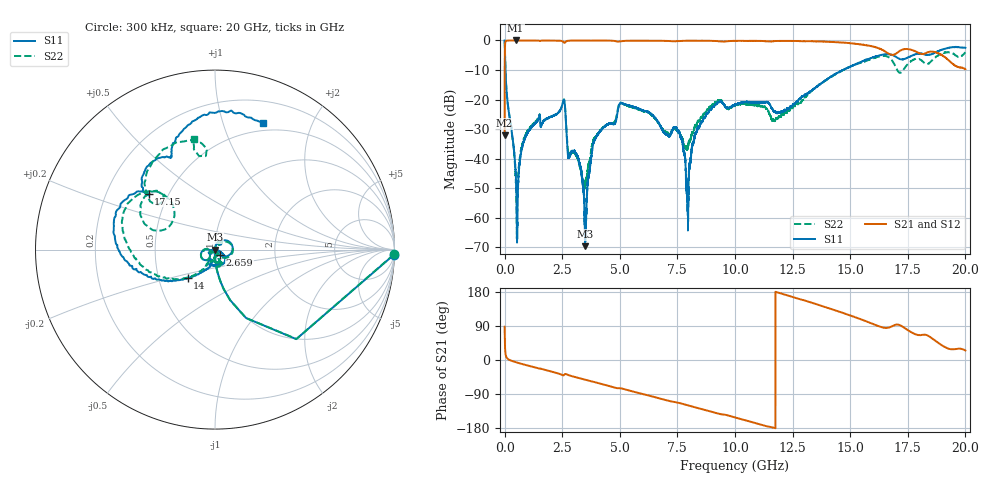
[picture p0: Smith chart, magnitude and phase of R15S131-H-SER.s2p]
!{R15S131}
!Johanson Technology Inc.
!www.johansontechnology.com
!Test Board Conditions:
!Substrate Type  RO4350B
!Substrate Thickness  20 mil
!Substrate Dk  3.66
!TL Type: GCPW
!TL Trace Width  34 mil
!TL Gap  10 mil
!Electrode orientation  Horizontal
!DUT TOPOLOGY	SERIES
!Mounting Pad LxW  26x52 mil
! Created Sat Feb  6 14:11:45 2021
# hz S ma R 50
! 2 Port Network Data from SP1.SP block
! freq  magS11  angS11  magS21  angS21  magS12  angS12  magS22  angS22
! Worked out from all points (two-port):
!   20001 points, 300 kHz to 20 GHz, reference 50 ohm
!   highest |S21| = 0.00 dB at 477.3 MHz (marker M1); lowest = -32.2 dB at 300 kHz (marker M2)
!   |S21| within 3 dB of the highest: 12.21 MHz to 16.35 GHz (16.34 GHz wide, 200 % of centre); 17.31 GHz to 17.57 GHz (265 MHz wide, 1.52 % of centre)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
!   lowest |S11| = -69.6 dB at 3.491 GHz (marker M3), VSWR 1.00, Z = 50 + j0.0294 ohm
!   |S11| at or under -10 dB: 36.21 MHz to 14.67 GHz (14.63 GHz wide, 199 % of centre); 14.66745 GHz to 14.67174 GHz (4.29 MHz wide, 0.0292 % of centre); 14.6865 GHz to 14.69163 GHz (5.126 MHz wide, 0.0349 % of centre)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
!   |S22| runs from -67.1 to 0.0 dB; largest |S21 - S12| = 0.018
!   S11 on the Smith chart (normalised r, x): 300 kHz: 6, -70; 2.659 GHz: 1.06, -0.07; 14 GHz: 0.70, -0.23; 17.15 GHz: 0.39, +0.32; 20 GHz: 0.42, +1.36
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300000  0.9976 -1.6  0.02468 87.8  0.02476 88.3  0.9963 -1.6
1.063e8  0.1103 -84.8  0.9932 4.9  0.9931 4.9  0.1107 -85.1
4.773e8  0.006006 -94.9  0.9998 -5.7  0.9985 -5.7  0.005338 -102.5
1.4343e9  0.0442 68.0  0.997 -21.6  0.9976 -21.5  0.04702 66.8
2.5313e9  0.08965 30.3  0.9604 -40.2  0.9607 -40.2  0.09019 22.9
2.6593e9  0.04347 -47.1  0.9548 -37.0  0.9557 -37.0  0.04651 -52.8
2.7973e9  0.0105 14.9  0.9906 -40.3  0.991 -40.3  0.01199 -7.2
3.3343e9  0.006049 46.7  0.9971 -49.5  0.9967 -49.5  0.005863 5.5
3.4913e9  0.0003301 117.0  0.997 -52.1  0.9977 -52.0  0.00364 -75.6
3.9093e9  0.02058 -140.5  0.9947 -58.3  0.9941 -58.4  0.02223 -136.2
5.0293e9  0.0872 -144.0  0.9647 -74.3  0.965 -74.3  0.08789 -146.2
6.6673e9  0.04148 177.1  0.9907 -100.4  0.9908 -100.4  0.04081 175.3
7.5943e9  0.02758 -160.1  0.9769 -113.8  0.978 -113.7  0.02706 -159.5
7.9473e9  0.001905 93.2  0.9878 -119.5  0.9889 -119.5  0.01583 -108.4
8.5753e9  0.04203 -26.6  0.9888 -129.7  0.9875 -129.7  0.05009 -68.9
1.00003e10  0.08219 -73.0  0.9839 -151.6  0.9833 -151.5  0.07909 -63.6
1.16863e10  0.0629 -117.5  0.9724 -178.8  0.9734 -178.7  0.04496 -90.0
1.33343e10  0.1427 -119.3  0.9711 151.2  0.9718 151.1  0.1415 -122.6
1.39993e10  0.2194 -134.1  0.9506 137.9  0.9517 137.9  0.2192 -134.6
1.66673e10  0.5808 156.4  0.5998 85.3  0.5839 85.7  0.522 143.5
1.71483e10  0.4844 139.8  0.6658 92.1  0.655 92.2  0.2844 146.8
2e10  0.7504 69.2  0.327 25.1  0.3218 25.2  0.6284 100.6
